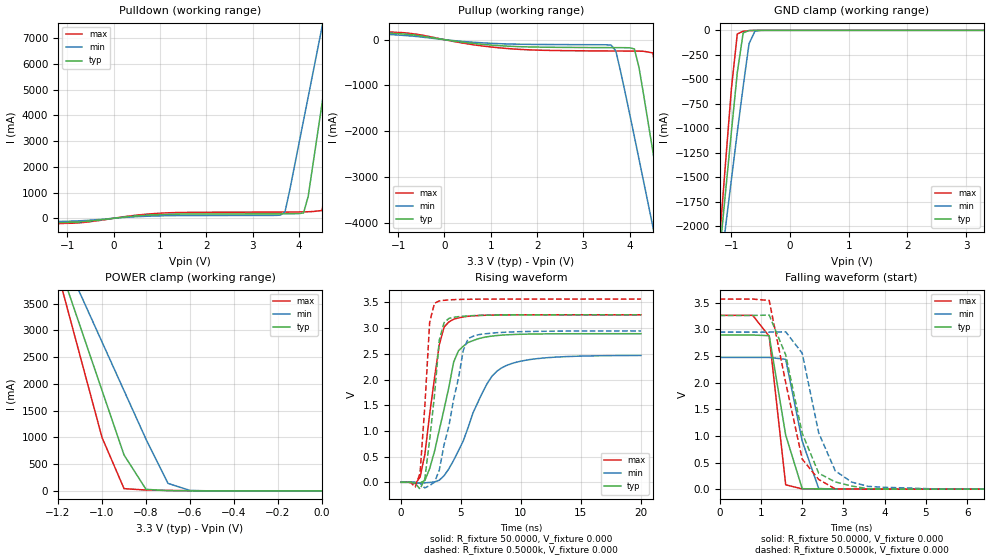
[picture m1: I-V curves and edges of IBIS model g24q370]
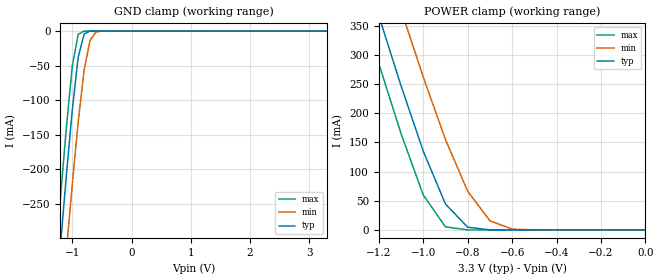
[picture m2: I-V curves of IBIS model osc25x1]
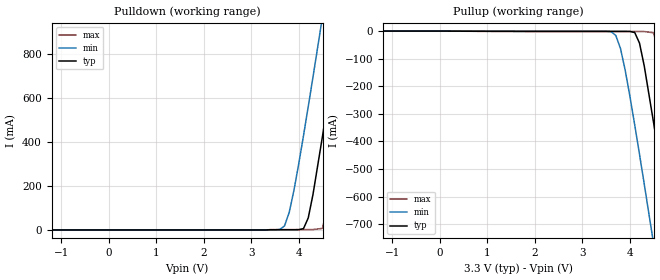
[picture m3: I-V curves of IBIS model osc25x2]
|   National Semiconductor Corporation
|   Interface Products Group
|   IBIS Model of DP83848 AspenPHY
|   48L LQFP Package
[IBIS Ver]   4.2
[Comment char]  |_char
[File name]   dp83848ksq.ibs
[File Rev]   1.1
[Date]   9/07/2010
[Source]   File originated at National Semiconductor Corporation.
   Interface Group/Analog Division. All models created with
   Spectre s2ibis simulations by Sida Zhang.
   Originally Created on 5/25/2006 by Sida Zhang, modified
   on 9/01/2010 by Peggy Alavi
[Notes]
   Rev 0.1 The file does not have TD+/TD- and RD+/RD- models
   due to the IBIS modeling limitations and design complexity.
   Rev 1.1 removes model selector. Model selector included a
   production test mode which is not available in the final
   product.
Begin IBIS Parser Results
| Do NOT edit this section manually!
Checking ...\dp83848jsq.ibs for IBIS 4.2 Compatibility...
WARNING - Model osc25x1: POWER Clamp : Typical value never becomes zero
WARNING - Model osc25x1: POWER Clamp : Minimum value never becomes zero
WARNING - Model osc25x1: POWER Clamp : Maximum value never becomes zero
Errors  : 0
Warnings: 3
File Passed
| End IBIS Parser Results
[Disclaimer]
(C) Copyright National Semiconductor Corporation 2010
   All rights reserved
   National Semiconductor Corporation hereby grants
the user of this IBIS model a non-exclusive, nontransferable
license to use this IBIS model under the following terms.
Before using this IBIS model, the user should read this
license.  If the user does not accept these terms,  the
IBIS model should be returned to National within 30 days.
   The user is granted this license only to use the
IBIS model and is not granted rights to sell, load, rent,
lease or license the IBIS model in whole or in part, or in
modified form to anyone other than user. User may modify
the IBIS model to suit its specific applications but rights
to derivative works and such modifications shall belong to
National.
   This IBIS model is provided on an "AS IS" basis and
National makes absolutely no warranty with respect to the
information contained herein.NATIONAL DISCLAIMS AND CUSTOMER
WAIVES ALL WARRANTIES, EXPRESS OR IMPLIED, INCLUDING
WARRANTIES OF MERCHANTABILITY OR FITNESS FOR A PARTICULAR
PURPOSE. The entire risk as to quality and performance is
with the Customer. ACCORDINGLY, IN NO EVENT SHALL THE
COMPANY BE LIABLE FOR ANY DAMAGES, WHETHER IN CONTRACT OR
TORT,INCLUDING ANY LOST PROFITS OR OTHER INCIDENTAL,
CONSEQUENTIAL, EXEMPLARY, OR PUNITIVE DAMAGES ARISING OUT
OF THE USE OR APPLICATION OF THE IBIS model provided in
this package.Further, National reserves the right to make
changes without notice to any product herein to improve
reliability, function, or design. National does not convey
any license under patent rights or any other intellectual
property rights, including those of third parties.
   National is not obligated to provide maintenance or support
for the licensed IBIS model.
[Copyright]   Copyright 2010, National Semiconductor, All Rights Reserved
[Component]   DP83848KSQ
[Manufacturer]  National Semiconductor Corporation
[Package]
|   typ   min   max
R_pkg   0.166   0.084   0.206
L_pkg   2.146n   1.025n   2.756n
C_pkg   0.077p   0.064p   0.088p
[Pin]   signal_name   model_name   R_pin   L_pin   C_pin
1   IOVDD33   POWER   0.20255   2.71780n   0.08735p
2   TX_CLK   g24q370   0.18067   2.37180n   0.07865p
3   TX_EN   g24q370   0.16766   2.14420n   0.07865p
4   TXD_0   g24q370   0.15753   1.99400n   0.06964p
5   TXD_1   g24q370   0.15231   1.92170n   0.06597p
6   TXD_2   g24q370   0.15266   1.93830n   0.06597p
7   TXD_3   g24q370   0.15721   2.02430n   0.06709p
8   RESERVED   NC   0.16414   2.13130n   0.06817p
9   RESERVED   NC   0.17487   2.30030n   0.07337p
10   RESERVED   NC   0.18743   2.51510n   0.08425p
11   RD-   NC   0.19121   2.55280n   0.08842p
12   RD+   NC   0.17578   2.26510n   0.08842p
13   AGND   GND   0.08381   1.02479n   0.08556p
14   TD-   NC   0.15196   1.89970n   0.08010p
15   TD+   NC   0.14507   1.80550n   0.06415p
16   PFBIN1   NC   0.14451   1.80320n   0.06641p
17   AGND   GND   0.15053   1.90440n   0.06641p
18   AVDD33   POWER   0.15750   2.00510n   0.07358p
19   PFBOUT   NC   0.17203   2.21300n   0.08623p
20   RBIAS   NC   0.18865   2.49100n   0.08623p
21   LED_SPEED   g24q370   0.18534   2.47560n   0.08596p
22   LED_LINK   g24q370   0.17739   2.32280n   0.07726p
23   RESET_N   g24q370   0.16445   2.10790n   0.07726p
24   MDIO   g24q370   0.15450   1.96000n   0.06578p
25   MDC   g24q370   0.14971   1.88380n   0.06578p
26   IOVDD33   POWER   0.15100   1.90170n   0.06587p
27   X2   osc25x2   0.15758   1.99420n   0.07013p
28   X1   osc25x1   0.16920   2.17150n   0.08808p
29   DGND   GND   0.09399   1.17744n   0.08808p
30   PFBIN2   NC   0.20112   2.70480n   0.08643p
31   RX_CLK   g24q370   0.20441   2.71850n   0.08615p
32   RX_DV   g24q370   0.18801   2.43970n   0.08615p
33   CRS/LED_CFG   g24q370   0.17380   2.22640n   0.07622p
34   RX_ER/MDIX_EN   g24q370   0.16329   2.08270n   0.07021p
35   COL/PHYAD0   g24q370   0.15844   2.01460n   0.06676p
36   RXD_0/PHYAD1   g24q370   0.15877   2.02240n   0.06676p
37   RXD_1/PHYAD2   g24q370   0.16413   2.10210n   0.07106p
38   RXD_2/PHYAD3   g24q370   0.17519   2.26280n   0.07759p
39   RXD_3/PHYAD4   g24q370   0.18965   2.48100n   0.08826p
40   IOGND   GND   0.20587   2.75580n   0.08826p
[Diff_pin]   inv_pin   vdiff   tdelay_typ   tdelay_min   tdelay_max
| The '+' pin is Diff_pin and the '-' pin is the inv_pin
12   11   0.100   0 0 0
15   14   0.100   0 0 0
| Models and submodels in the file (3): g24q370 (I/O), osc25x1 (Input), osc25x2 (Output)
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|   Model g24q370
[Model]   g24q370
Model_type   I/O
Polarity   Non-Inverting
Enable   Active-High
Vinl = 0.8000V
Vinh = 2.0000V
Vmeas = 1.5000V
C_comp   1.0640pF   1.0620pF   1.0670pF
[Temperature Range]   25.0000   0.1250k   -40.0000
[Voltage Range]   3.3000V   3.0000V   3.6000V
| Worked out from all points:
|   slope of the pulldown table from 0 to 0.495 V, typ, clamps not added: 5.31 ohm
|   slope of the pullup table from 0 to 0.495 V, typ, clamps not added: 7.25 ohm
|   GND clamp passes 1 mA (typ) near -0.64 V on its own axis
|   POWER clamp passes 1 mA (typ) near -0.54 V on its own axis
|   rising waveform, R_fixture 50.0000, V_fixture 0.000: 20-80 % time 1.6ns typ, 2.8ns min, 1.1ns max; typ from 0 V to 2.89 V
|   rising waveform, R_fixture 0.5000k, V_fixture 0.000: 20-80 % time 833ps typ, 1.56ns min, 573ps max; typ from 0 V to 3.26 V
|   falling waveform, R_fixture 50.0000, V_fixture 0.000: 20-80 % time 452ps typ, 464ps min, 281ps max; typ from 2.89 V to 0 V
|   falling waveform, R_fixture 0.5000k, V_fixture 0.000: 20-80 % time 659ps typ, 611ps min, 580ps max; typ from 3.26 V to 0 V
[Pulldown]
| voltage   I(typ)   I(min)   I(max)
-3.3V     -160.5mA   -118.3mA   -200.7mA
-900mV    -153.7mA   -111mA     -192.4mA
1.1V      151.8mA    98.11mA    206.2mA
3.6V      174.1mA    121.6mA    241.2mA
3.7V      174.7mA    254.1mA    242mA
4.1V      208.2mA    3.809A     248.7mA
4.2V      852.2mA    4.721A     254.3mA
4.5V      4.477A     7.457A     302mA
4.7V      6.898A     9.283A     2.796A
4.9V      9.321A     11.11A     5.87A
5.1V      11.75A     12.94A     8.947A
6.6V      30.05A     26.73A     32.17A
[Pullup]
| voltage   I(typ)   I(min)   I(max)
-3.3V     188.1mA    165.2mA    206.9mA
-900mV    123.6mA    93.95mA    153.1mA
1.3V      -138.1mA   -91.87mA   -188.7mA
3.6V      -174.3mA   -119.7mA   -247.2mA
3.7V      -174.6mA   -248.3mA   -247.7mA
4.1V      -202.3mA   -2.118A    -249.5mA
4.2V      -607mA     -2.608A    -250.6mA
4.5V      -2.447A    -4.087A    -288.9mA
4.7V      -3.699A    -5.076A    -1.602A
4.9V      -4.956A    -6.068A    -3.14A
5.1V      -6.215A    -7.061A    -4.687A
6.6V      -15.68A    -14.52A    -16.34A
[GND_clamp]
| voltage   I(typ)   I(min)   I(max)
-3.3V     -15.47A    -12.9A     -18.37A
-1.2V     -2.269A    -2.494A    -2.116A
-1.1V     -1.647A    -2.005A    -1.349A
-1V       -1.031A    -1.519A    -592.6mA
-900mV    -430.7mA   -1.039A    -37.49mA
-800mV    -26.32mA   -572.9mA   -9.444mA
-700mV    -1.926mA   -136.4mA   -3.598mA
-600mV    -247.7uA   -8.119mA   -648.8uA
-400mV    -1.571uA   -27.47uA   -1.62uA
3.3V      22.02pA    3.648uA    15.2pA
[POWER_clamp]
| voltage   I(typ)   I(min)   I(max)
-3.3V     29.64A     23.74A     36.19A
-1.2V     4.29A      4.604A     4.058A
-1.1V     3.083A     3.693A     2.528A
-1V       1.877A     2.784A     997.8mA
-900mV    671.8mA    1.874A     42.61mA
-800mV    29.37mA    964.9mA    16.3mA
-700mV    5.409mA    140.5mA    9.688mA
-600mV    1.864mA    8.479mA    4.466mA
0V        22.02pA    589.3pA    18.15pA
[Ramp]
| variable   typ   min   max
dV/dt_r   1.7348/1.6680n   1.4811/3.0471n   1.9560/1.1060n
dV/dt_f   1.8068/1.8411n   1.5594/3.2593n   2.0132/1.2189n
R_load = 50.0000
[Rising Waveform]
R_fixture = 50.0000
V_fixture = 0.000
V_fixture_min = 0.000
V_fixture_max = 0.000
| time   V(typ)   V(min)   V(max)
0s        121pV      6.465nV    36.64pV
1.6ns     -12.04mV   -15.26mV   96.9mV
2ns       34.22mV    -11.2mV    543.1mV
2.4ns     268mV      -3.569mV   1.326V
3.2ns     1.016V     39.7mV     2.674V
4ns       1.85V      262mV      3.12V
4.8ns     2.559V     613.5mV    3.2V
7.2ns     2.832V     1.925V     3.252V
8.4ns     2.864V     2.227V     3.257V
20ns      2.891V     2.468V     3.26V
[Rising Waveform]
R_fixture = 0.5000k
V_fixture = 0.000
V_fixture_min = 0.000
V_fixture_max = 0.000
| time   V(typ)   V(min)   V(max)
0s        130pV      7.171nV    38.79pV
1.2ns     -20.26mV   28.89uV    -92.41mV
1.6ns     -134.2mV   -21.16mV   180.7mV
2ns       72.06mV    -111.1mV   1.492V
2.4ns     825.8mV    -63.59mV   3.114V
2.8ns     1.692V     781.9uV    3.485V
3.2ns     2.765V     233.9mV    3.529V
3.6ns     3.107V     729.7mV    3.542V
5.6ns     3.239V     2.796V     3.562V
20ns      3.259V     2.945V     3.566V
[Falling Waveform]
R_fixture = 50.0000
V_fixture = 0.000
V_fixture_min = 0.000
V_fixture_max = 0.000
| time   V(typ)   V(min)   V(max)
0s        2.891V     2.471V     3.26V
800ps     2.891V     2.471V     3.26V
1.2ns     2.878V     2.471V     2.867V
1.6ns     1.014V     2.436V     81.31mV
2ns       8.918mV    903.1mV    5.147mV
2.4ns     3.412mV    11.78mV    4.297mV
20ns      2.471uV    23.79uV    19.15uV
[Falling Waveform]
R_fixture = 0.5000k
V_fixture = 0.000
V_fixture_min = 0.000
V_fixture_max = 0.000
| time   V(typ)   V(min)   V(max)
0s        3.259V     2.945V     3.566V
1.2ns     3.265V     2.946V     3.539V
1.6ns     2.519V     2.952V     1.996V
2ns       1.048V     2.55V      564.1mV
2.4ns     298.8mV    1.056V     181.6mV
2.8ns     136.3mV    345.2mV    4.978mV
3.2ns     58.01mV    132.1mV    1.436mV
3.6ns     8.285mV    52.25mV    931.6uV
5.2ns     739.4uV    5.88mV     479.6uV
20ns      3.35uV     19.65uV    13.62uV
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|   Model osc25x1
[Model]   osc25x1
Model_type   Input
Polarity   Inverting
Enable   Active-High
Vinl = 0.8000V
Vinh = 2.0000V
C_comp   1.0000pF   1.0000pF   1.0000pF
[Temperature Range]   25.0000   0.1250k   -40.0000
[Voltage Range]   3.3000V   3.0000V   3.6000V
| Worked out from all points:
|   GND clamp passes 1 mA (typ) near -0.72 V on its own axis
|   POWER clamp passes 1 mA (typ) near -0.72 V on its own axis
[GND_clamp]
| voltage   I(typ)   I(min)   I(max)
-3.3V     -2.622A    -2.694A    -2.579A
-1.3V     -414.8mA   -523mA     -346.4mA
-1.2V     -310.3mA   -419.8mA   -240.9mA
-1.1V     -208.9mA   -318.8mA   -139.7mA
-1V       -114.1mA   -221.5mA   -50.66mA
-900mV    -37.58mA   -131mA     -4.515mA
-800mV    -4.019mA   -56.03mA   -47.48uA
-700mV    -108.1uA   -13.33mA   -2.355uA
-600mV    -3.685uA   -1.282mA   -1.753uA
-400mV    -1.001uA   -4.899uA   -1.167uA
3.3V      8.25uA     7.477uA    9.629uA
[POWER_clamp]
| voltage   I(typ)   I(min)   I(max)
-3.3V     3.1A       3.186A     3.05A
-1.3V     490.5mA    618.5mA    409.7mA
-1.2V     366.9mA    496.4mA    284.9mA
-1.1V     247mA      377mA      165.2mA
-1V       135mA      261.9mA    59.9mA
-900mV    44.44mA    154.8mA    5.346mA
-800mV    4.759mA    66.25mA    66.21uA
-700mV    135.7uA    15.76mA    12.92uA
-600mV    12.33uA    1.522mA    12.26uA
-500mV    9.553uA    95.08uA    11.96uA
0V        8.25uA     6.563uA    10.5uA
|   Model osc25x2
[Model]   osc25x2
Model_type   Output
Polarity   Inverting
Enable   Active-High
Vmeas = 1.5000V
C_comp   1.0000pF   1.0000pF   1.0000pF
[Temperature Range]   25.0000   0.1250k   -40.0000
[Voltage Range]   3.3000V   3.0000V   3.6000V
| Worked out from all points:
|   slope of the pullup table from 0 to 0.495 V, typ, clamps not added: 1.19 kohm
[Pulldown]
| voltage   I(typ)   I(min)   I(max)
-3.3V     0A         0A         0A
3.6V      1.099mA    2.318mA    1.555mA
3.7V      1.103mA    18.37mA    1.56mA
3.8V      1.11mA     80.08mA    1.567mA
4.1V      6.217mA    428mA      1.603mA
4.2V      54.57mA    559.8mA    1.639mA
4.5V      425.9mA    967.9mA    7.417mA
4.7V      707.9mA    1.245A     200.5mA
4.9V      996mA      1.525A     486.1mA
5.1V      1.287A     1.806A     783.4mA
5.3V      1.58A      2.089A     1.085A
6.6V      3.503A     3.939A     3.076A
[Pullup]
| voltage   I(typ)   I(min)   I(max)
-3.3V     0A         0A         0A
3.6V      -1.081mA   -2.06mA    -1.527mA
3.7V      -1.083mA   -15.55mA   -1.53mA
3.8V      -1.086mA   -63.14mA   -1.534mA
4.1V      -5.367mA   -340.7mA   -1.543mA
4.2V      -43.48mA   -446.6mA   -1.551mA
4.5V      -335.7mA   -775mA     -6.395mA
4.7V      -559.6mA   -998.5mA   -156mA
4.9V      -788.6mA   -1.224A    -379.2mA
5.1V      -1.02A     -1.451A    -612.3mA
5.3V      -1.253A    -1.678A    -849mA
6.6V      -2.784A    -3.17A     -2.413A
[Ramp]
| variable   typ   min   max
dV/dt_r   1.7737/0.4988n   1.5328/0.7567n   1.9870/0.3615n
dV/dt_f   1.8364/0.4766n   1.5967/0.7630n   2.0404/0.3438n
R_load = 10.0000k
